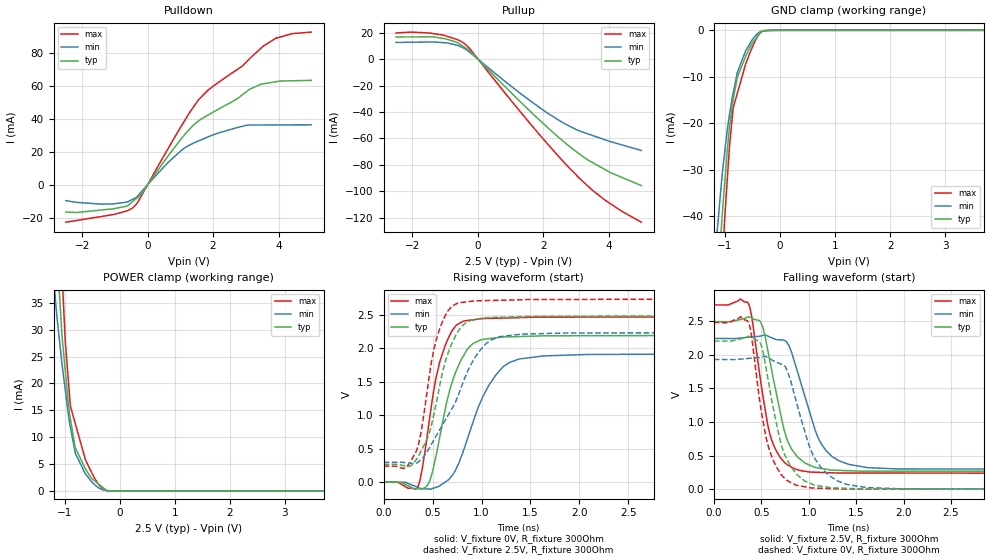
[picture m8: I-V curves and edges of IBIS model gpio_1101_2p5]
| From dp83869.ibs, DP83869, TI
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|   gpio_1101_2p5 Model
[Model]   gpio_1101_2p5
Model_type   I/O
Polarity   Non-Inverting
Enable   Active-Low
Vinl = 0.7
Vinh = 1.7
Vmeas = 1.25
Vref = 0
Cref = 2pF
Rref = 100000
|   typ   min   max
C_comp   1.246pF   1.092pF   1.323pF
| Where Nom  PVT is Nominal Process, 2.5V,  27C
|   Fast PVT is Strong Process,  2.75V, -40C
|   Slow PVT is Weak Process,   2.25V, 125C
[Voltage Range]   2.5   2.25   2.75
|Junction Temperature
[Temperature Range]   27   125   -40
[Pullup Reference]   2.5   2.25   2.75
[Pulldown Reference]   -0   0   0
[Power Clamp Reference]   2.5   2.25   2.75
[GND Clamp Reference]   0   0   0
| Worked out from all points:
|   slope of the pulldown table from 0 to 0.375 V, typ, clamps not added: 35.6 ohm
|   slope of the pullup table from 0 to 0.375 V, typ, clamps not added: 39.3 ohm
|   GND clamp passes 1 mA (typ) near -0.39 V on its own axis
|   POWER clamp passes 1 mA (typ) near -0.35 V on its own axis
|   falling waveform, V_fixture 2.5V, R_fixture 300Ohm: 20-80 % time 209ps typ, 269ps min, 177ps max; typ from 2.49 V to 0.264 V
|   rising waveform, V_fixture 0V, R_fixture 300Ohm: 20-80 % time 228ps typ, 322ps min, 188ps max; typ from 0 V to 2.2 V
|   rising waveform, V_fixture 2.5V, R_fixture 300Ohm: 20-80 % time 227ps typ, 393ps min, 179ps max; typ from 0.264 V to 2.49 V
|   falling waveform, V_fixture 0V, R_fixture 300Ohm: 20-80 % time 217ps typ, 276ps min, 184ps max; typ from 2.2 V to 0 V
[Pulldown]
|   Voltage   I(typ)   I(min)   I(max)
-2.5V     -16.58mA   -9.648mA   -22.72mA
-1.054V   -14.63mA   -11.63mA   -18.14mA
-624.7mV  -12.95mA   -10.53mA   -15.84mA
-441.9mV  -10.01mA   -8.731mA   -13.94mA
-232.5mV  -6.635mA   -5.179mA   -8.27mA
1.039V    28.07mA    20.9mA     35.83mA
1.554V    38.63mA    26.51mA    51.42mA
1.845V    42.22mA    28.94mA    57.28mA
2.907V    54.73mA    35.46mA    72.12mA
3.128V    57.97mA    36.19mA    76.63mA
3.937V    62.49mA    36.24mA    89.03mA
5V        63.25mA    36.3mA     92.52mA
[GND Clamp]
|   Voltage   I(typ)   I(min)   I(max)
-2.5V     -325.5mA   -278mA     -374.2mA
-1.151V   -58.23mA   -45.14mA   -72.46mA
-1.062V   -42.41mA   -32.96mA   -53.35mA
-1.027V   -36.66mA   -28.83mA   -45.97mA
-1.003V   -32.97mA   -26.33mA   -40.67mA
-915mV    -20.93mA   -18.18mA   -25mA
-847.5mV  -14.88mA   -13.5mA    -16.71mA
-770.2mV  -10.08mA   -9.023mA   -13.47mA
-624.7mV  -5.69mA    -4.486mA   -7.365mA
-464.4mV  -2.203mA   -1.455mA   -2.671mA
-358.7mV  -487uA     -330.5uA   -624.1uA
5V        0A         0A         0A
[Pullup]
|   Voltage   I(typ)   I(min)   I(max)
-2.5V     16.85mA    12.69mA    19.89mA
-2.038V   16.89mA    12.84mA    20.55mA
-1.293V   16.72mA    12.97mA    19.14mA
-624.7mV  12.72mA    10.59mA    14.92mA
-425.4mV  9.413mA    8.367mA    12.24mA
-232.5mV  6.21mA     4.984mA    7.654mA
979.2mV   -24.36mA   -19.66mA   -30.06mA
1.926V    -46.95mA   -37.29mA   -58.26mA
2.572V    -61.3mA    -47.66mA   -76.36mA
3.125V    -72.19mA   -54.52mA   -90.62mA
3.937V    -84.28mA   -61.44mA   -107.7mA
5V        -95.76mA   -69.14mA   -123.5mA
[POWER Clamp]
|   Voltage   I(typ)   I(min)   I(max)
-2.5V     383.1mA    300.3mA    465.8mA
-1.265V   71.43mA    49.25mA    97.27mA
-1.162V   48.95mA    35.07mA    69.59mA
-1.083V   35.05mA    27.13mA    48.53mA
-1.045V   28.71mA    23.46mA    40.27mA
-931.5mV  16.22mA    14.27mA    20.59mA
-894.7mV  13.4mA     11.9mA     15.8mA
-802.5mV  7.998mA    6.976mA    12.43mA
-624.2mV  4.162mA    3.227mA    5.916mA
-348.9mV  1.007mA    388uA      837.2uA
-117mV    1.734uA    21.08uA    18.09uA
5V        0A         0A         0A
[Ramp]
R_load = 300
|   typ   min   max
dV/dt_r   1.31978/2.26312e-10   1.15396/3.19812e-10   1.48539/1.86564e-10
dV/dt_f   1.33571/2.08168e-10   1.16705/2.69502e-10   1.50173/1.7604e-10
[Falling Waveform]
V_fixture = 2.5V
V_fixture_min = 2.25V
V_fixture_max = 2.75V
R_fixture = 300Ohm
C_fixture = 0F
|   Time   V(typ)   V(min)   V(max)
0s        2.49V      2.241V     2.739V
366.4ps   2.563V     2.258V     2.759V
491.4ps   2.49V      2.276V     1.632V
567.8ps   2.077V     2.277V     963.1mV
621.9ps   1.684V     2.244V     686.3mV
742.2ps   874.6mV    2.213V     402.3mV
860.2ps   519mV      1.848V     297.7mV
1.122ns   310.9mV    702.1mV    249.2mV
1.425ns   274.1mV    367.6mV    240.4mV
5ns       264mV      295.5mV    236.6mV
[Rising Waveform]
V_fixture = 0V
V_fixture_min = 0V
V_fixture_max = 0V
R_fixture = 300Ohm
C_fixture = 0F
|   Time   V(typ)   V(min)   V(max)
0s        103.8uV    187.3uV    101.1uV
349.4ps   -104.1mV   -80.73mV   -71.57mV
393.6ps   -104.4mV   -99.61mV   191.1mV
465.2ps   -708.4uV   -106.7mV   905.3mV
573.1ps   670.4mV    -56.99mV   1.796V
682.9ps   1.415V     67.31mV    2.221V
813.6ps   1.884V     459.8mV    2.408V
1.083ns   2.148V     1.467V     2.45V
1.388ns   2.178V     1.843V     2.462V
5ns       2.2V       1.923V     2.476V
[Rising Waveform]
V_fixture = 2.5V
V_fixture_min = 2.25V
V_fixture_max = 2.75V
R_fixture = 300Ohm
C_fixture = 0F
|   Time   V(typ)   V(min)   V(max)
0s        264mV      295.5mV    236.6mV
224.7ps   237.5mV    288.8mV    212mV
332.6ps   333.2mV    282.2mV    459.7mV
455ps     683.8mV    481.6mV    1.471V
538.9ps   1.193V     694.2mV    2.138V
637.2ps   1.841V     945.1mV    2.512V
755.4ps   2.239V     1.273V     2.678V
943.8ps   2.439V     1.888V     2.713V
1.195ns   2.468V     2.177V     2.722V
5ns       2.49V      2.24V      2.739V
[Falling Waveform]
|Gnd
V_fixture = 0V
V_fixture_min = 0V
V_fixture_max = 0V
R_fixture = 300Ohm
C_fixture = 0F
|   Time   V(typ)   V(min)   V(max)
0s        2.202V     1.928V     2.477V
363.9ps   2.272V     1.943V     2.488V
488.5ps   2.175V     1.958V     1.274V
558.7ps   1.737V     1.963V     721.3mV
637.2ps   1.132V     1.902V     398.4mV
755ps     489.4mV    1.817V     151.2mV
864.1ps   238.4mV    1.331V     60.26mV
1.071ns   56.95mV    441.6mV    16.01mV
1.411ns   12.08mV    67.4mV     3.612mV
5ns       103.5uV    185.3uV    100.3uV
